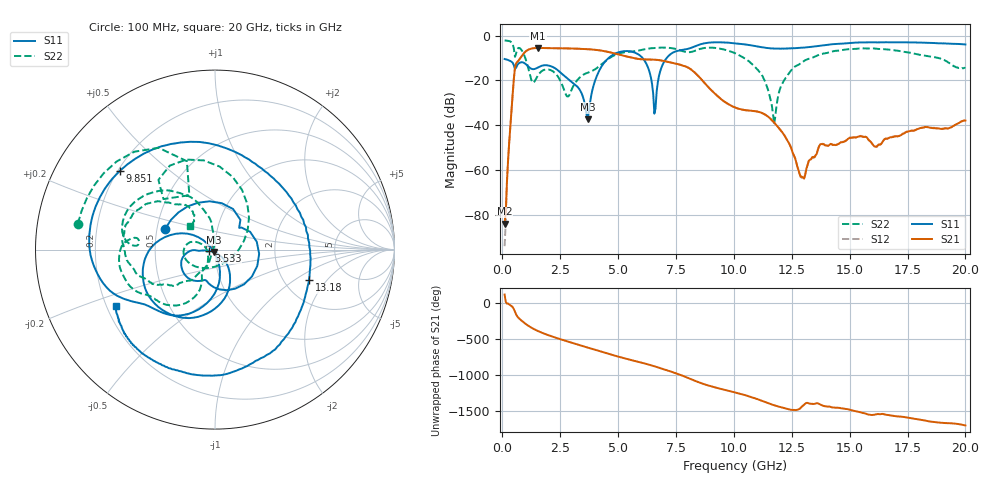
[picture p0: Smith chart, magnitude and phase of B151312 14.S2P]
!  2-Port S-parameters saved by WinCal
! VAR MeasName=S-Parameters (CALIBRATED_DATA) read from VNA (N5244A)
! VAR MeasDate=12/8/2015 5:44:38 PM
! VAR NAME=B151312 14
! VAR FILENAME=B151312 14.S2P
! VAR DATE=12/8/2015 5:44:38 PM
! VAR PHYS_PORTS=1,2
# Hz S DB R 50
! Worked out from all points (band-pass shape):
!   401 points, 100 MHz to 20 GHz, reference 50 ohm
!   highest |S21| = -5.53 dB at 1.543 GHz (marker M1); lowest = -83.8 dB at 100 MHz (marker M2)
!   |S21| within 3 dB of the highest: 882.9 MHz to 5.071 GHz (4.188 GHz wide, 141 % of centre)
!   lowest |S11| = -37.3 dB at 3.682 GHz (marker M3), VSWR 1.03, Z = 49.5 - j1.24 ohm
!   |S11| at or under -10 dB: start of sweep to 4.593 GHz; 6.057 GHz to 7.1 GHz (1.043 GHz wide, 15.9 % of centre)
!   |S22| runs from -39.5 to -2.2 dB; largest |S21 - S12| = 0.0015
!   S11 on the Smith chart (normalised r, x): 100 MHz: 0.55, +0.14; 3.533 GHz: 0.93, -0.01; 9.851 GHz: 0.21, +0.35; 13.18 GHz: 2.72, -1.33; 20 GHz: 0.24, -0.25
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1e8  -10.45 157.5  -83.80 119.9  -93.80 93.2  -2.19 169.3
5.975e8  -14.33 39.7  -12.35 -158.1  -12.35 -158.1  -7.91 135.6
9.955e8  -12.56 -73.8  -7.22 73.7  -7.22 73.7  -10.11 54.8
1.54275e9  -14.22 -116.2  -5.53 -29.9  -5.53 -30.0  -17.73 -129.1
2.63725e9  -17.60 -177.9  -5.70 -156.8  -5.70 -156.8  -23.36 160.9
3.43325e9  -25.91 -174.4  -5.95 124.4  -5.94 124.4  -17.91 -120.1
3.53275e9  -29.06 -171.5  -5.99 114.8  -5.99 114.7  -17.25 -120.5
3.682e9  -37.31 -113.0  -6.07 100.3  -6.07 100.3  -16.57 -119.2
4.876e9  -8.00 -107.5  -8.04 -14.8  -8.03 -14.9  -8.64 -123.3
6.02025e9  -9.57 173.5  -10.58 -111.6  -10.58 -111.6  -6.39 -149.4
6.5675e9  -34.79 164.6  -10.74 -161.2  -10.73 -161.2  -5.56 -162.1
6.7665e9  -18.02 -77.2  -10.94 178.3  -10.94 178.4  -5.41 -167.0
8.3585e9  -4.60 -153.0  -16.94 -9.4  -16.91 -9.7  -6.63 176.7
9.851e9  -3.25 140.2  -31.03 -150.9  -31.06 -151.1  -7.07 132.1
1.005e10  -3.44 131.2  -32.06 -167.0  -32.08 -167.3  -7.84 126.4
1.119425e10  -5.19 76.3  -34.40 78.7  -34.43 78.7  -17.34 97.1
1.17415e10  -5.78 50.5  -38.72 14.3  -38.77 14.5  -39.51 153.2
1.29355e10  -5.42 -7.2  -62.82 -5.3  -63.41 -6.5  -12.04 -134.7
1.318425e10  -5.18 -18.0  -57.67 47.7  -57.63 50.7  -10.53 -137.4
1.338325e10  -5.00 -25.8  -54.25 34.7  -54.25 36.8  -9.87 -141.6
1.67165e10  -3.02 -113.7  -45.50 -124.1  -45.19 -124.8  -6.29 152.9
2e10  -3.96 -150.4  -37.85 92.5  -37.85 91.5  -14.41 136.6
